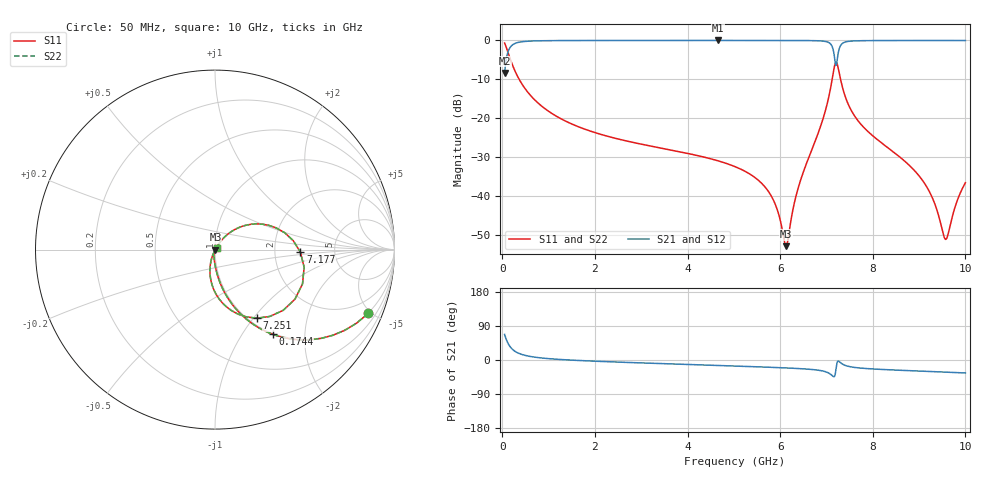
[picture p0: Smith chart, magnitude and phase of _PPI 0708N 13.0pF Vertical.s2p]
! S-Parameter data specifications (vertical orientation):
! Substrate: 40-mil Rogers 3003C, Substrate thickness, H=1.016mm, Dielectric constant, Er=3, Conductor thickness, T_mtl=0.043mm, Loss Tangent, Tand=0.003
! PCB Mounting Pad Footprint: Pad width, PadW=2.54mm , Pad length, PadL=0.51mm , Pad gap, PadG (edge-to-edge)=0.71mm , Reference planes=1.73mm apart
! Created Tue Jan 16 08:52:01 2018
# GHz S MA R 50
! 2 Port Network Data from SP1.SP block
! freq  magS11  angS11  magS21  angS21  magS12  angS12  magS22  angS22
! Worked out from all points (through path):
!   801 points, 50 MHz to 10 GHz, reference 50 ohm
!   highest |S21| = -0.02 dB at 4.652 GHz (marker M1); lowest = -8.4 dB at 50 MHz (marker M2)
!   group delay of S21, straight-line fit = 12.7 ps
!   lowest |S11| = -52.8 dB at 6.132 GHz (marker M3), VSWR 1.00, Z = 50.2 - j0.0804 ohm
!   |S11| at or under -10 dB: 364.9 MHz to 7.123 GHz (6.758 GHz wide, 181 % of centre); 7.305 GHz to end of sweep
!   |S22| runs from -52.8 to -0.7 dB; largest |S21 - S12| = 0
!   S11 on the Smith chart (normalised r, x): 50 MHz: 0.99, -4.81; 174.4 MHz: 0.99, -1.38; 7.177 GHz: 2.81, -0.11; 7.251 GHz: 1.09, -1.04; 10 GHz: 1.02, +0.02
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0.05  0.9244 -22.6  0.3812 67.4  0.3812 67.4  0.9244 -22.6
0.174375  0.5711 -55.8  0.8206 34.2  0.8206 34.2  0.5711 -55.8
0.3485  0.3294 -71.9  0.9439 18.0  0.9439 18.0  0.3294 -71.9
0.721625  0.1677 -82.7  0.9854 7.1  0.9854 7.1  0.1677 -82.7
1.716625  0.07507 -91.2  0.9964 -1.7  0.9964 -1.7  0.07507 -91.2
3.370812  0.04217 -97.9  0.998 -9.2  0.998 -9.2  0.04217 -97.9
4.651875  0.02862 -101.9  0.9982 -14.4  0.9982 -14.4  0.02862 -101.9
5.025  0.02403 -102.6  0.9981 -15.9  0.9981 -15.9  0.02403 -102.6
5.746375  0.01156 -100.2  0.9979 -19.0  0.9979 -19.0  0.01156 -100.2
5.9205  0.007208 -94.1  0.9978 -19.8  0.9978 -19.8  0.007208 -94.1
6.131938  0.002294 -20.4  0.9974 -20.9  0.9974 -20.9  0.002294 -20.4
6.380687  0.01226 53.3  0.9966 -22.4  0.9966 -22.4  0.01226 53.3
6.691625  0.04068 56.8  0.9932 -25.1  0.9932 -25.1  0.04068 56.8
7.089625  0.2458 35.1  0.8988 -37.7  0.8988 -37.7  0.2458 35.1
7.176687  0.4761 -1.8  0.5893 -42.5  0.5893 -42.5  0.4761 -1.8
7.251313  0.4483 -58.5  0.6753 -2.9  0.6753 -2.9  0.4483 -58.5
7.350812  0.2433 -89.3  0.9208 -11.2  0.9208 -11.2  0.2433 -89.3
7.599563  0.1091 -104.8  0.9848 -19.5  0.9848 -19.5  0.1091 -104.8
8.345812  0.04118 -111.9  0.996 -25.8  0.996 -25.8  0.04118 -111.9
9.129375  0.01431 -109.5  0.9969 -29.8  0.9969 -29.8  0.01431 -109.5
9.564687  0.002819 -40.0  0.9968 -32.0  0.9968 -32.0  0.002819 -40.0
10  0.01493 43.4  0.9963 -34.2  0.9963 -34.2  0.01493 43.4
